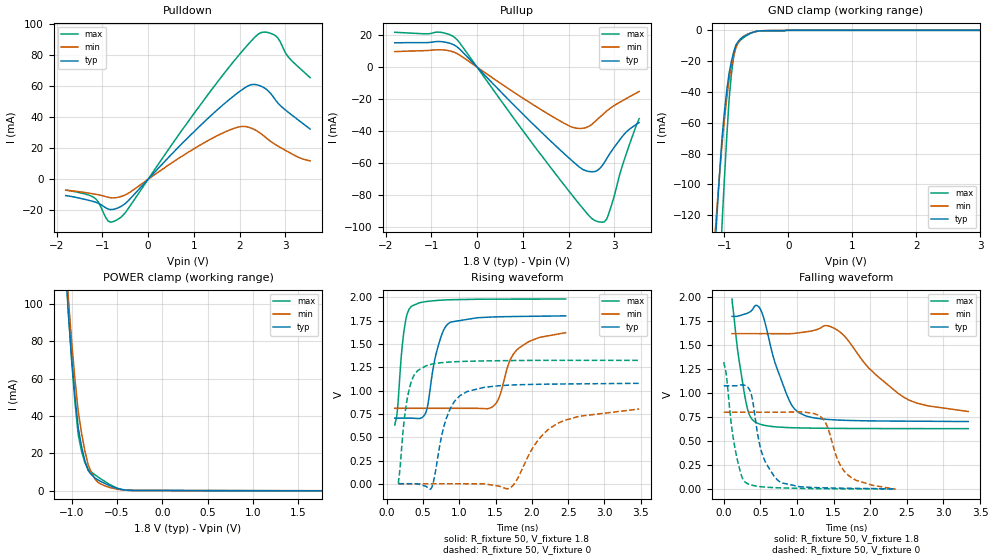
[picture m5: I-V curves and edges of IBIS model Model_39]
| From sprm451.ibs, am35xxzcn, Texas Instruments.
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| Model based on original model for BC1833DV40CTPBFZP18LL_7LM_X50
|   Sub model LL_7LM_X50_PU_ON_1P8
[model]   Model_39
|[Description]  1.8V-I/O-PU-X
|[Input Load]   PU
|[Output Drive]
|Voltage   1.8V
|Mode   I/O
Model_type   I/O
Polarity   Non-Inverting
Enable   Active-Low
Vinl =  0.63V
Vinh =  1.17V
Cref =  15pF
Rref =  100.0000M
Vref =  0V
Vmeas =  0.9
C_comp   2.232809p   2.073051p   2.295852p
[Model Spec]
Vinl   0.63V   0.567V   0.693V
Vinh   1.17V   1.053V   1.287V
[Temperature Range]   25   125   -40
[Voltage Range]   1.8   1.62   1.98
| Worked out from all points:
|   slope of the pulldown table from 0 to 0.27 V, typ, clamps not added: 31.4 ohm
|   slope of the pullup table from 0 to 0.27 V, typ, clamps not added: 33.4 ohm
|   GND clamp passes 1 mA (typ) near -0.53 V on its own axis
|   POWER clamp passes 1 mA (typ) near -0.49 V on its own axis
|   rising waveform, R_fixture 50, V_fixture 1.8: 20-80 % time 169ps typ, 257ps min, 93ps max; typ from 0.705 V to 1.8 V
|   rising waveform, R_fixture 50, V_fixture 0: 20-80 % time 226ps typ, 476ps min, 132ps max; typ from 0.003 V to 1.08 V
|   falling waveform, R_fixture 50, V_fixture 1.8: 20-80 % time 284ps typ, 648ps min, 154ps max; typ from 1.8 V to 0.705 V
|   falling waveform, R_fixture 50, V_fixture 0: 20-80 % time 213ps typ, 260ps min, 144ps max; typ from 1.08 V to 0.003 V
[POWER_clamp]
-1.8V     842.3mA    869.2mA    912.6mA
-1.073V   123.5mA    130.8mA    128.8mA
-1.036V   94.69mA    102.8mA    96.31mA
-1V       70.7mA     79.63mA    69.41mA
-963.6mV  50.3mA     59.44mA    47.21mA
-927.3mV  33.48mA    42.27mA    29.73mA
-890.9mV  23.56mA    30.73mA    21mA
-818.2mV  10.72mA    13.8mA     11.42mA
-709.1mV  5.624mA    4.312mA    7.236mA
-527.3mV  1.606mA    1.01mA     1.915mA
-381.8mV  142.3uA    117.5uA    127.8uA
1.764V    -143.5uA   -80.17uA   -225.9uA
[Pulldown]
-1.8V     -10.49mA   -6.992mA   -6.878mA
-1.145V   -14.77mA   -9.642mA   -12.54mA
-872.7mV  -19.18mA   -11.58mA   -26.88mA
-600mV    -17.64mA   -11.15mA   -24.61mA
1.636V    48.04mA    29.95mA    67.37mA
2.073V    58.21mA    34.18mA    83.2mA
2.291V    61.28mA    32.65mA    90.41mA
2.455V    60.33mA    29.78mA    94.55mA
2.618V    57.37mA    25.94mA    94.82mA
2.782V    51.43mA    22.55mA    92.84mA
3.055V    43.59mA    17.92mA    79.47mA
3.545V    32.43mA    11.97mA    65.61mA
[Pullup]
-1.8V     15.27mA    9.71mA     21.85mA
-818.2mV  16.05mA    10.88mA    21.94mA
-490.9mV  13.72mA    9.223mA    18.66mA
1.036V    -30.45mA   -20.11mA   -41.15mA
2.018V    -57.22mA   -36.91mA   -78.08mA
2.345V    -64.63mA   -38.19mA   -89.73mA
2.618V    -65.01mA   -33.11mA   -96.69mA
2.782V    -59.96mA   -28.87mA   -97.07mA
2.836V    -57.32mA   -27.51mA   -95.25mA
3V        -50.25mA   -24.09mA   -80.87mA
3.218V    -42.03mA   -20.43mA   -58.16mA
3.545V    -34.78mA   -15.26mA   -32.29mA
[GND_clamp]
-1.8V     -697.8mA   -553.3mA   -1.259A
-1.145V   -140.7mA   -131.7mA   -248.4mA
-1.109V   -115.2mA   -111.7mA   -203.4mA
-1.036V   -69.7mA    -74.11mA   -126mA
-1V       -53.27mA   -58.3mA    -96.66mA
-927.3mV  -28.09mA   -31.91mA   -45.55mA
-890.9mV  -20.27mA   -23.39mA   -28.66mA
-854.5mV  -14.02mA   -16.45mA   -16.77mA
-818.2mV  -9.337mA   -11.08mA   -9.893mA
-672.7mV  -3.466mA   -3.226mA   -3.973mA
-18.18mV  0A         0A         0A
3.6V      0A         0A         0A
[Ramp]
dV/dt_f 0.72574948/0.29709567n 0.53575278/0.67541976n 0.88790778/0.16185442n
dV/dt_r 0.68043054/0.22625319n 0.51236198/0.47394452n 0.81151986/0.1318087n
R_load = 50
[Rising Waveform]
R_fixture = 50
V_fixture = 1.8
V_fixture_min = 1.62
V_fixture_max = 1.98
109.1ps   705.3mV    810mV      631.5mV
145ps     705.3mV    810mV      785.1mV
234.8ps   705.3mV    810mV      1.63V
339.8ps   704.7mV    810mV      1.903V
536.6ps   763.6mV    810mV      1.952V
704.9ps   1.469V     810mV      1.966V
880.2ps   1.734V     810mV      1.973V
1.441ns   1.787V     818.2mV    1.979V
1.791ns   1.794V     1.434V     1.98V
2.467ns   1.8V       1.62V      1.98V
[Rising Waveform]
R_fixture = 50
V_fixture = 0
V_fixture_min = 0
V_fixture_max = 0
159.9ps   2.802mV    1.768mV    3.967mV
242.7ps   2.811mV    1.771mV    709.1mV
315.5ps   2.355mV    1.77mV     1.037V
541.1ps   -25.69mV   1.767mV    1.265V
631.1ps   -10.89mV   1.768mV    1.284V
861ps     783.7mV    1.766mV    1.306V
1.109ns   990mV      1.467mV    1.314V
1.692ns   1.058V     -45.14mV   1.321V
2.358ns   1.07V      649.3mV    1.324V
3.481ns   1.078V     802.6mV    1.324V
[Falling Waveform]
R_fixture = 50
V_fixture = 1.8
V_fixture_min = 1.62
V_fixture_max = 1.98
113.1ps   1.8V       1.62V      1.98V
194.2ps   1.803V     1.62V      1.419V
306.6ps   1.829V     1.62V      894mV
444.5ps   1.915V     1.62V      694.1mV
532.2ps   1.815V     1.62V      670mV
859.4ps   986.4mV    1.62V      643.2mV
1.023ns   798.3mV    1.629V     639.5mV
1.484ns   724.1mV    1.685V     634.6mV
2.465ns   709.4mV    955.4mV    632.1mV
3.338ns   705.3mV    810mV      631.5mV
[Falling Waveform]
R_fixture = 50
V_fixture = 0
V_fixture_min = 0
V_fixture_max = 0
0s        1.078V     802.6mV    1.324V
147.5ps   1.077V     802.6mV    449.4mV
287.7ps   1.082V     802.6mV    77.57mV
379.2ps   977.5mV    802.6mV    44.14mV
477.4ps   511.9mV    802.6mV    30.17mV
540.9ps   333mV      802.6mV    24.88mV
784.9ps   68.27mV    802.6mV    14.78mV
1.327ns   16.54mV    753.3mV    6.633mV
1.659ns   11.67mV    176.5mV    4.985mV
2.346ns   2.802mV    1.768mV    3.967mV
